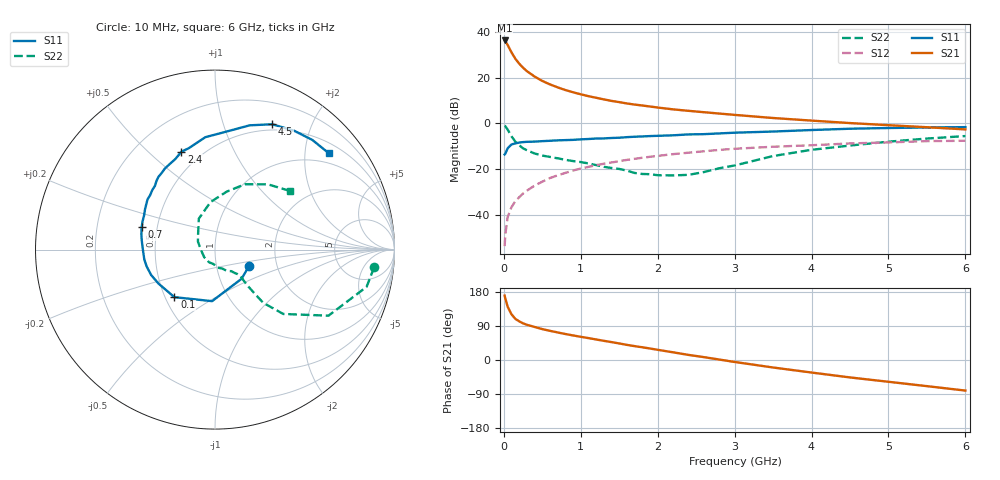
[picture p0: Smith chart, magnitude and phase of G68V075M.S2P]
! SIEMENS Small Signal Semiconductors
! BFG193
! Si NPN RF Bipolar Junction Transistor in SOT223
! VCE = 8 V  IC = 75 mA
! Common Emitter S-Parameters:  August  1996
# GHz  S  MA  R  50
!  f  S11  S21  S12  S22
! GHz  MAG  ANG  MAG  ANG  MAG  ANG  MAG  ANG
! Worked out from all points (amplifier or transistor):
!   36 points, 10 MHz to 6 GHz, reference 50 ohm
!   highest |S21| = 36.2 dB at 10 MHz (marker M1)
!   |S21| within 3 dB of that: start of sweep to 65.4 MHz
!   unconditionally stable (mu >= 1): 371.9 MHz to 2.357 GHz
!   at 250 MHz: K = 0.94, MSG = 27.4 dB, |S12| = -30.6 dB
!   at 1.4 GHz: K = 1.05, MAG = 12.1 dB, |S12| = -17.0 dB
!   at 6 GHz: K = 0.89, MSG = 2.5 dB, |S12| = -7.6 dB
!   S11 on the Smith chart (normalised r, x): 10 MHz: 1.44, -0.27; 100 MHz: 0.56, -0.34; 700 MHz: 0.41, +0.12; 2.4 GHz: 0.39, +0.64; 4.5 GHz: 0.43, +1.47; 6 GHz: 0.74, +2.55
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0.01  0.2108 -24.9  64.73 170.0  0.0021 81.5  0.8919 -6.4
0.02  0.2199 -47.6  62 162.0  0.0039 77.7  0.8698 -13.8
0.05  0.2877 -93.2  51.37 140.3  0.0091 71.6  0.7318 -30.2
0.1  0.3485 -130.5  35.46 120.5  0.015 66.4  0.523 -43.3
0.15  0.3674 -149.0  25.72 108.5  0.0202 66.7  0.4003 -47.8
0.2  0.383 -158.3  20.18 102.0  0.0246 69.2  0.3347 -48.0
0.25  0.3922 -166.2  16.43 96.7  0.0296 69.9  0.2859 -47.9
0.3  0.3977 -172.0  13.84 92.9  0.0342 70.7  0.2601 -47.9
0.4  0.4014 -179.6  10.55 87.2  0.044 70.7  0.2212 -46.7
0.5  0.4111 173.0  8.469 81.5  0.0537 69.7  0.1992 -46.1
0.6  0.4188 168.4  7.111 77.0  0.0644 68.6  0.186 -47.3
0.7  0.4273 163.1  6.128 72.7  0.0738 67.2  0.1735 -49.4
0.9  0.4384 154.4  4.789 64.8  0.0939 63.6  0.151 -52.7
1.1  0.4579 146.9  3.941 57.8  0.1129 60.3  0.1342 -61.4
1.3  0.4716 140.1  3.351 50.6  0.1324 56.1  0.1132 -68.8
1.6  0.5024 130.5  2.73 39.9  0.1604 49.3  0.0935 -87.5
2.2  0.5511 113.6  2.031 20.3  0.214 35.8  0.0735 -145.4
2.4  0.5766 108.9  1.885 13.5  0.2301 31.5  0.0756 -173.7
3.5  0.6662 83.2  1.315 -19.8  0.3104 4.5  0.1945 117.6
4.5  0.7674 65.5  1.019 -46.0  0.3664 -15.6  0.3294 78.6
5.5  0.817 48.4  0.827 -69.0  0.4121 -39.1  0.4681 51.0
6  0.8313 40.1  0.742 -80.7  0.4185 -52.6  0.5312 37.9
